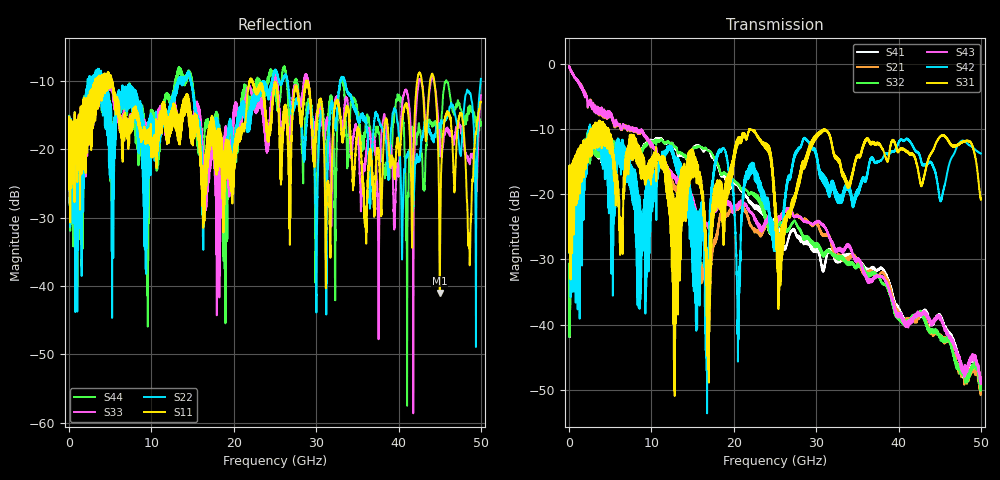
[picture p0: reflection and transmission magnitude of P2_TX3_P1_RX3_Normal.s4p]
!Keysight Technologies,N5225A,MY51441389,A.10.49.11
!Date: Monday, July 08, 2019 13:20:09
!Correction: S11(Full 4 Port(1,2,3,4))
!S12(Full 4 Port(1,2,3,4))
!S13(Full 4 Port(1,2,3,4))
!S14(Full 4 Port(1,2,3,4))
!S21(Full 4 Port(1,2,3,4))
!S22(Full 4 Port(1,2,3,4))
!S23(Full 4 Port(1,2,3,4))
!S24(Full 4 Port(1,2,3,4))
!S31(Full 4 Port(1,2,3,4))
!S32(Full 4 Port(1,2,3,4))
!S33(Full 4 Port(1,2,3,4))
!S34(Full 4 Port(1,2,3,4))
!S41(Full 4 Port(1,2,3,4))
!S42(Full 4 Port(1,2,3,4))
!S43(Full 4 Port(1,2,3,4))
!S44(Full 4 Port(1,2,3,4))
!S4P File: Measurements: <S11,S12,S13,S14>,
!<S21,S22,S23,S24>,
!<S31,S32,S33,S34>,
!<S41,S42,S43,S44>:
# Hz S  dB  R 50
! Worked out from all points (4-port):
!   5000 points, 10 MHz to 50 GHz, reference 50 ohm
!   strongest paths, dB at 10 MHz, 12.51 GHz, 25.01 GHz, 37.51 GHz, 50 GHz:
!     S31: -19.3, -19.5, -20.5, -12.2, -20.9
!     S42: -19.4, -12.9, -27.4, -15.0, -13.8
!     S43: -0.4, -16.7, -25.3, -32.6, -48.6
!     S32: -33.3, -12.4, -24.5, -32.5, -50.0
!     S21: -0.4, -17.7, -26.4, -32.4, -50.5
!     S41: -33.0, -12.2, -24.2, -31.5, -49.4
!   lowest |S11| = -41.0 dB at 45.02 GHz (marker M1), VSWR 1.02, Z = 49.2 + j0.283 ohm
!   |S11| at or under -10 dB: 5.216 GHz to 21.93 GHz (16.72 GHz wide, 123 % of centre); 22.25 GHz to 28.82 GHz (6.574 GHz wide, 25.7 % of centre); 28.92 GHz to 42.27 GHz (13.35 GHz wide, 37.5 % of centre)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
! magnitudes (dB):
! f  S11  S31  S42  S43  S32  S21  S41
! 10 MHz  -17.7  -19.3  -19.4  -0.4  -33.3  -0.4  -33.0
! 15.03 GHz  -19.4  -13.7  -22.7  -20.8  -13.1  -21.5  -13.0
! 16.84 GHz  -18.6  -35.7  -33.2  -25.0  -13.3  -38.5  -13.3
! 22 GHz  -9.8  -10.1  -17.0  -22.7  -19.8  -24.6  -21.2
! 25.52 GHz  -17.8  -34.7  -27.2  -23.4  -24.1  -23.9  -25.6
! 45.02 GHz  -41.0  -11.2  -20.9  -38.8  -41.9  -41.9  -38.5
! 50 GHz  -13.1  -20.9  -13.8  -48.6  -50.0  -50.5  -49.4
